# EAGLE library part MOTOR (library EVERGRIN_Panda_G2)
Motor
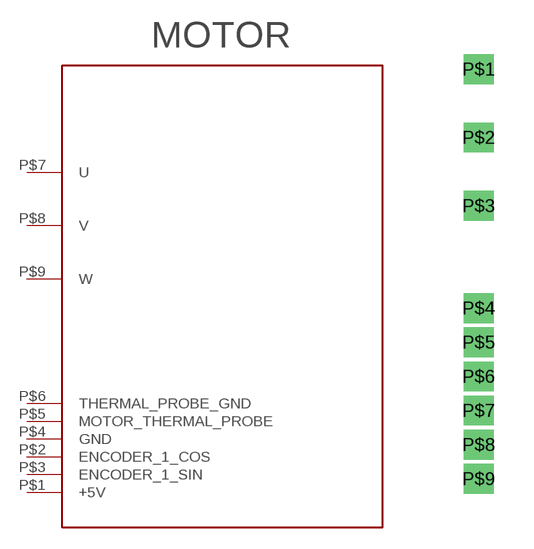
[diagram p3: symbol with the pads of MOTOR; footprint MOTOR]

Designator prefix -

## MOTOR  [MOTOR]
P$1  +5V
P$2  ENCODER_1_COS
P$3  ENCODER_1_SIN
P$4  GND
P$5  MOTOR_THERMAL_PROBE
P$6  THERMAL_PROBE_GND
P$7  U
P$8  V
P$9  W

## Footprint MOTOR (pad centres in mm)
drill 0.6 square: P$1 -1.27,24.13; P$2 -1.27,21.59; P$3 -1.27,19.05; P$4 -1.27,15.24; P$5 -1.27,13.97; P$6 -1.27,12.7; P$7 -1.27,11.43; P$8 -1.27,10.16; P$9 -1.27,8.89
